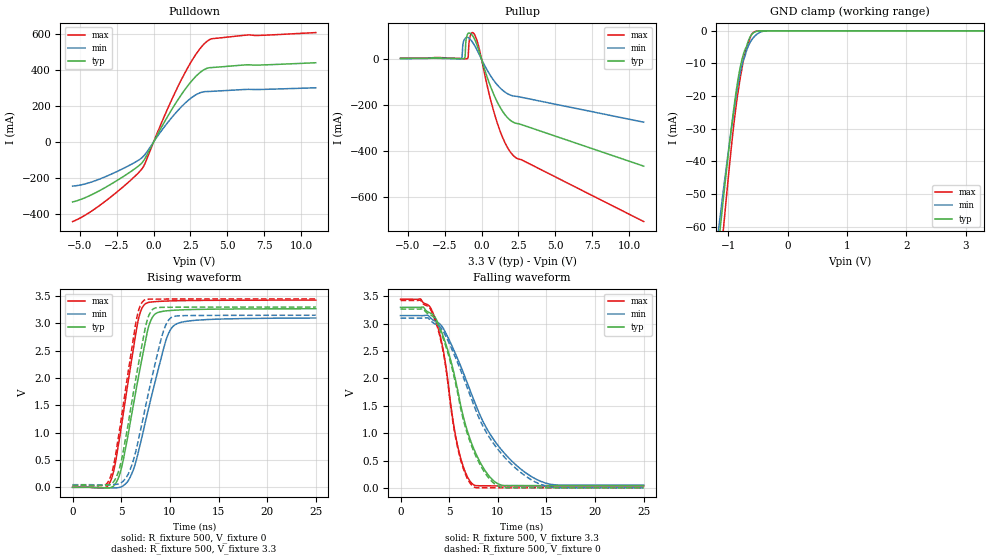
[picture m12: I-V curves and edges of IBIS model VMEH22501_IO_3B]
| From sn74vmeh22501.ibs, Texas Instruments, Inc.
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[Model]   VMEH22501_IO_3B
Model_type  I/O
Vinh =   1.7
Vinl =   1.6
Enable   Active-Low
Vref =   0
Rref =   500
Cref =   50p
Vmeas =   1.5
| variable   typ   min   max
C_comp   10.25pF   9.60pF   11.37pF
| C_pullup   28.09pF   12.01pF   55.01pF
| C_pulldown   12.89pF   9.82pF   16.24pF
| C_tri-state   10.25pF   9.60pF   11.37pF
[Temperature Range]   40   100   0
| Ambient temperature   25   85   0
[Voltage range]   3.3   3.15   3.45
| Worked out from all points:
|   slope of the pulldown table from 0 to 0.495 V, typ, clamps not added: 6.54 ohm
|   slope of the pullup table from 0 to 0.495 V, typ, clamps not added: 5.03 ohm
|   GND clamp passes 1 mA (typ) near -0.60 V on its own axis
|   rising waveform, R_fixture 500, V_fixture 0: 20-80 % time 2.05ns typ, 2.54ns min, 1.81ns max; typ from 0 V to 3.27 V
|   falling waveform, R_fixture 500, V_fixture 3.3: 20-80 % time 2.96ns typ, 5.05ns min, 1.84ns max; typ from 3.3 V to 0.04 V
|   rising waveform, R_fixture 500, V_fixture 3.3: 20-80 % time 1.94ns typ, 2.33ns min, 1.75ns max; typ from 0.04 V to 3.3 V
|   falling waveform, R_fixture 500, V_fixture 0: 20-80 % time 2.96ns typ, 4.99ns min, 1.85ns max; typ from 3.27 V to 0 V
[GND Clamp]
| VMEH22501_IO_3B
|   Voltage   I(typ)   I(min)   I(max)
-5.5V     -906.2mA   -787.6mA   -1.055A
-1.165V   -65.88mA   -61.35mA   -77.74mA
-1.14V    -61.55mA   -57.61mA   -72.67mA
-1.105V   -55.56mA   -52.42mA   -65.66mA
-1.075V   -50.49mA   -48.04mA   -59.74mA
-920mV    -25.91mA   -26.62mA   -31.16mA
-820mV    -13.34mA   -15mA      -17.12mA
-760mV    -8.243mA   -9.962mA   -10.69mA
-705mV    -5.308mA   -6.938mA   -5.973mA
-575mV    -606.8uA   -2.078mA   -468.8uA
-325mV    -628.4nA   -12.08uA   -399nA
3.3V      155.7pA    15.27nA    -3.387nA
[Pulldown]
| VMEH22501_IO_3B
|   Voltage   I(typ)   I(min)   I(max)
-5.5V     -333.1mA   -244.9mA   -441.7mA
-3.315V   -254.4mA   -194.5mA   -331.2mA
-1.755V   -176.1mA   -134.9mA   -226.9mA
-785mV    -115.4mA   -87mA      -148.4mA
-575mV    -90.54mA   -68.32mA   -117.3mA
890mV     132.5mA    100.3mA    172.6mA
1.9V      264mA      195.7mA    347.5mA
2.85V     361.7mA    259.9mA    482.9mA
3.625V    407.7mA    278.7mA    557.2mA
3.995V    411.9mA    280.1mA    572mA
6.35V     426.9mA    290.8mA    591.8mA
11V       438.3mA    299.6mA    605.5mA
[Pullup]
| VMEH22501_IO_3B
|   Voltage   I(typ)   I(min)   I(max)
-5.5V     4.043mA    3.022mA    5.145mA
-1.41V    2.882mA    2.3mA      3.583mA
-1.185V   2.699mA    83.77mA    3.172mA
-1.12V    12.73mA    90.4mA     3.063mA
-970mV    106.7mA    95.96mA    2.974mA
-905mV    113.3mA    94.87mA    14.86mA
-800mV    113.8mA    89.14mA    94.22mA
-575mV    99.56mA    70.79mA    115.5mA
-225mV    46.57mA    30.03mA    62.32mA
1.045V    -182.9mA   -109.4mA   -272.6mA
2.1V      -271.4mA   -158.3mA   -414.6mA
11V       -464.2mA   -273.2mA   -705.2mA
[Ramp]
| VMEH22501_IO_3B
| variable   typ   min   max
dV/dt_r   1.97/2.05E-09   1.86/2.57E-09   2.06/1.82E-09
dV/dt_f   1.96/2.98E-09   1.87/5.06E-09   2.05/1.87E-09
R_load = 500
[Rising Waveform]
| VMEH22501_IO_3B
R_fixture =   500
C_fixture =   0
L_fixture =   0
V_fixture =   0
V_fixture_min = 0
V_fixture_max = 0
|   Time   V(typ)   V(min)   V(max)
0s        233.4uV    1.149uV    793.7uV
3.945ns   -2.414mV   -8.219mV   133.9mV
4.85ns    241.6mV    484.6uV    929mV
5.87ns    1.128V     169.5mV    2.113V
6.77ns    2.02V      655.3mV    3.079V
7.455ns   2.648V     1.177V     3.356V
8.385ns   3.156V     1.865V     3.397V
9.675ns   3.23V      2.732V     3.41V
10.57ns   3.242V     2.98V      3.414V
24.99ns   3.268V     3.099V     3.426V
[Falling Waveform]
| VMEH22501_IO_3B
R_fixture =   500
C_fixture =   0
L_fixture =   0
V_fixture =   3.3
V_fixture_min = 3.15
V_fixture_max = 3.45
|   Time   V(typ)   V(min)   V(max)
0s        3.3V       3.15V      3.449V
2.065ns   3.3V       3.149V     3.454V
3.415ns   3.155V     3.061V     3.162V
4.45ns    2.739V     2.899V     2.463V
5.375ns   2.183V     2.561V     1.252V
5.95ns    1.721V     2.326V     705.5mV
7.43ns    758.6mV    1.653V     66.42mV
9.88ns    88.32mV    807.7mV    35.16mV
13.91ns   40.63mV    159.8mV    33.25mV
24.99ns   39.69mV    48.55mV    32.99mV
[Rising Waveform]
| VMEH22501_IO_3B
R_fixture =   500
C_fixture =   0
L_fixture =   0
V_fixture =   3.3
V_fixture_min = 3.15
V_fixture_max = 3.45
|   Time   V(typ)   V(min)   V(max)
0s        39.67mV    48.23mV    32.99mV
3.86ns    52.36mV    47.54mV    179mV
4.78ns    323.8mV    66.49mV    999.3mV
5.73ns    1.18V      248.1mV    2.133V
6.64ns    2.13V      767.7mV    3.138V
7.33ns    2.79V      1.337V     3.421V
8.2ns     3.251V     2.046V     3.445V
9.335ns   3.294V     2.856V     3.446V
10.17ns   3.296V     3.11V      3.447V
24.99ns   3.3V       3.15V      3.449V
[Falling Waveform]
| VMEH22501_IO_3B
R_fixture =   500
C_fixture =   0
L_fixture =   0
V_fixture =   0
V_fixture_min = 0
V_fixture_max = 0
|   Time   V(typ)   V(min)   V(max)
0s        3.27V      3.103V     3.427V
2.065ns   3.27V      3.102V     3.431V
3.41ns    3.12V      3.011V     3.136V
4.45ns    2.697V     2.843V     2.429V
5.36ns    2.14V      2.502V     1.236V
5.935ns   1.676V     2.26V      685.3mV
7.44ns    707.3mV    1.557V     29.25mV
9.875ns   46.96mV    735.4mV    1.175mV
13.88ns   718.3uV    105.1mV    806.3uV
24.99ns   245.9uV    243.7uV    796uV
